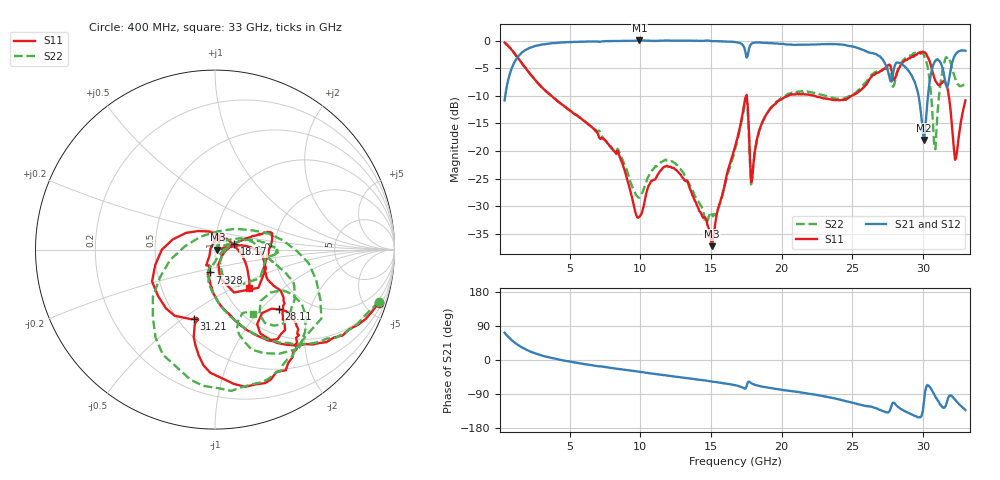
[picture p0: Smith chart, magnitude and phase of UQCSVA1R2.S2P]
!  Part Number  UQCSVA1R2  Mounting Orientation: Horizontal
!  Description: Ultra Low ESR Microwave capacitors
!  Application: Coupling, Bypass, Tuning, DC Block
!  Filters, Matching
# GHZ S DB R 50
! Freq  |S11|  S11 Ph  |S21|  S21 Ph  |S12|  S12 Ph  |S22|  S22 Ph
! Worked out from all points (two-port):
!   401 points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, 400 MHz to 33 GHz, reference 50 ohm
!   highest |S21| = 0.03 dB at 9.936 GHz (marker M1); lowest = -18.0 dB at 30.07 GHz (marker M2)
!   |S21| within 3 dB of the highest: 1.332 GHz to 17.51 GHz (16.17 GHz wide, 172 % of centre); 17.55 GHz to 27 GHz (9.449 GHz wide, 42.4 % of centre)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
!   lowest |S11| = -37.2 dB at 15.07 GHz (marker M3), VSWR 1.03, Z = 51.4 - j0.0574 ohm
!   |S11| at or under -10 dB: 3.711 GHz to 17.49 GHz (13.78 GHz wide, 130 % of centre); 17.52 GHz to 20.46 GHz (2.94 GHz wide, 15.5 % of centre); 22.31 GHz to 24.94 GHz (2.628 GHz wide, 11.1 % of centre)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
!   |S22| runs from -33.0 to -0.4 dB; largest |S21 - S12| = 0.0091
!   S11 on the Smith chart (normalised r, x): 400 MHz: 0.85, -6.17; 7.328 GHz: 0.91, -0.24; 18.17 GHz: 1.24, +0.08; 28.11 GHz: 1.45, -1.27; 31.21 GHz: 0.60, -0.55; 33 GHz: 1.31, -0.61
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0.4  -0.37 -18.1  -10.83 71.8  -10.84 71.7  -0.36 -17.7
2.356  -6.46 -69.0  -1.13 20.3  -1.12 20.5  -6.53 -68.9
5.861  -14.22 -97.6  -0.21 -9.7  -0.21 -9.8  -14.20 -99.6
7.328  -17.70 -103.0  -0.13 -17.6  -0.14 -17.6  -17.47 -107.2
9.936  -31.87 148.1  0.03 -31.0  0.02 -31.1  -28.45 -32.2
11.321  -23.93 80.2  -0.01 -37.9  -0.02 -38.1  -22.40 17.4
15.07  -37.21 -2.3  -0.09 -57.0  -0.10 -57.1  -31.56 54.2
16.7  -19.27 10.3  -0.25 -66.4  -0.26 -66.2  -19.81 32.9
17.434  -10.38 -20.2  -2.03 -75.7  -2.00 -75.0  -10.87 -11.6
17.841  -25.65 -44.2  -0.63 -61.0  -0.63 -61.0  -26.04 -36.7
18.167  -19.05 15.7  -0.33 -66.3  -0.34 -66.3  -19.18 18.0
19.471  -11.60 19.4  -0.51 -75.6  -0.47 -75.7  -11.45 8.7
22.161  -9.91 8.2  -0.72 -90.1  -0.71 -90.0  -9.38 -3.7
27.621  -4.31 -55.2  -6.57 -135.7  -6.57 -135.7  -5.43 -52.3
28.11  -6.24 -43.0  -4.03 -119.5  -4.09 -119.7  -6.25 -30.0
29.251  -2.87 -50.9  -6.57 -144.4  -6.58 -144.8  -2.55 -59.6
30.066  -2.11 -73.3  -17.98 -110.6  -17.66 -110.7  -2.63 -100.5
30.8  -6.73 -104.5  -3.98 -91.1  -4.01 -91.3  -19.39 137.1
31.207  -7.91 -107.0  -3.81 -116.6  -3.81 -116.1  -8.38 7.8
31.778  -9.27 -165.5  -7.92 -100.2  -7.90 -100.9  -2.93 -51.3
32.267  -21.59 77.4  -2.64 -104.6  -2.66 -105.1  -6.79 -74.5
33  -10.81 -48.2  -1.83 -132.0  -1.81 -131.9  -7.63 -59.7
